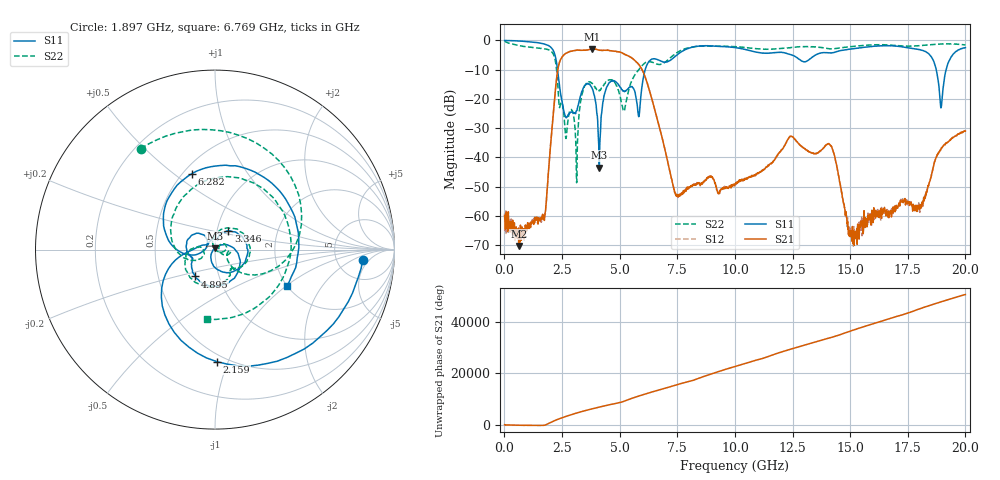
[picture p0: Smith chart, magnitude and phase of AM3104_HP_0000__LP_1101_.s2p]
!Created with skrf (http://scikit-rf.org).
# Hz S RI R 50.0
!freq ReS11 ImS11 ReS21 ImS21 ReS12 ImS12 ReS22 ImS22
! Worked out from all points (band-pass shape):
!   1601 points, 10 MHz to 20 GHz, reference 50 ohm
!   highest |S21| = -2.87 dB at 3.821 GHz (marker M1); lowest = -70.4 dB at 622.2 MHz (marker M2)
!   |S21| within 3 dB of the highest: 2.484 GHz to 5.506 GHz (3.022 GHz wide, 75.6 % of centre)
!   lowest |S11| = -43.5 dB at 4.12 GHz (marker M3), VSWR 1.01, Z = 49.8 + j0.645 ohm
!   |S11| at or under -10 dB: 2.305 GHz to 6.108 GHz (3.803 GHz wide, 90.4 % of centre); 18.74 GHz to 19.16 GHz (428.7 MHz wide, 2.26 % of centre)
!   |S22| runs from -48.7 to -0.2 dB; largest |S21 - S12| = 0.006
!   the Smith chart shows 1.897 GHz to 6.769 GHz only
!   S11 on the Smith chart (normalised r, x): 1.897 GHz: 9.23, -3.21; 2.159 GHz: 0.45, -0.91; 3.346 GHz: 1.13, +0.24; 4.895 GHz: 0.77, -0.24; 6.282 GHz: 0.55, +0.58; 6.769 GHz: 1.98, -1.02
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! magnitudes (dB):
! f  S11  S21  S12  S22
! 10 MHz  0.0  -59.9  -59.2  -0.2
! 622.2 MHz  -0.2  -70.4  -64.3  -1.7
! 1.897 GHz  -1.7  -46.4  -46.5  -3.1
! 2.159 GHz  -4.1  -21.5  -21.5  -5.4
! 2.671 GHz  -26.4  -4.4  -4.4  -33.6
! 3.146 GHz  -24.0  -3.3  -3.3  -48.1
! 3.346 GHz  -17.8  -3.4  -3.4  -19.2
! 3.821 GHz  -16.6  -2.9  -2.9  -14.8
! 4.12 GHz  -43.5  -3.3  -3.3  -17.1
! 4.895 GHz  -14.6  -3.8  -3.9  -15.8
! 5.82 GHz  -25.9  -8.1  -8.1  -10.1
! 6.282 GHz  -7.1  -16.8  -16.8  -7.3
! 6.682 GHz  -6.7  -28.4  -28.4  -8.2
! 6.769 GHz  -7.0  -31.0  -30.9  -8.2
! 7.494 GHz  -5.0  -52.7  -52.9  -4.1
! 10.01 GHz  -2.4  -49.2  -49.0  -2.1
! 13.34 GHz  -5.8  -38.5  -38.5  -2.2
! 14.2 GHz  -4.2  -36.5  -36.5  -2.9
! 15.03 GHz  -3.0  -67.0  -64.9  -2.1
! 16.68 GHz  -1.8  -60.7  -59.5  -1.5
! 18.95 GHz  -22.9  -37.0  -36.9  -1.2
! 20 GHz  -2.5  -31.0  -30.9  -1.5
